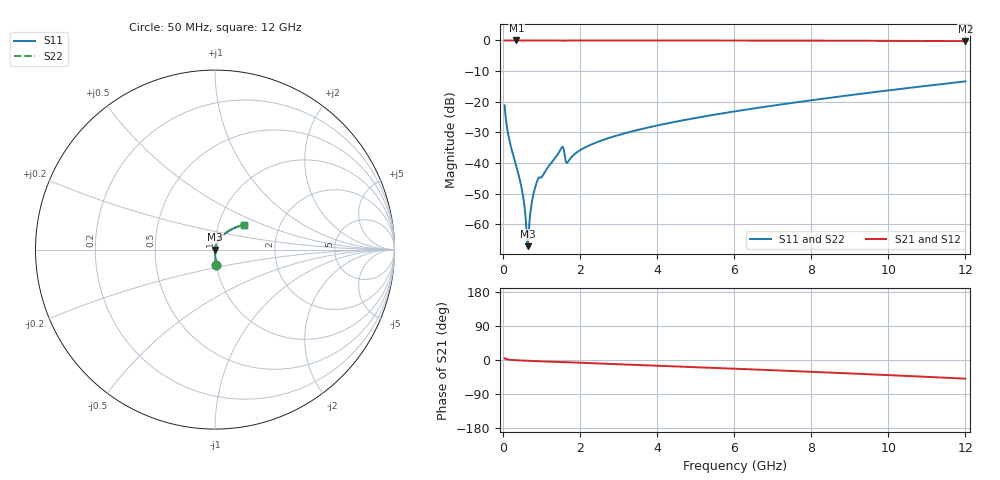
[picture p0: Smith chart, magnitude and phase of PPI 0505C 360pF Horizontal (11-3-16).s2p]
# MHz S MA R 50
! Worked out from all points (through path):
!   1601 points, 50 MHz to 12 GHz, reference 50 ohm
!   highest |S21| = 0.00 dB at 356.2 MHz (marker M1); lowest = -0.2 dB at 12 GHz (marker M2)
!   group delay of S21, straight-line fit = 11.4 ps
!   lowest |S11| = -67.1 dB at 647.5 MHz (marker M3), VSWR 1.00, Z = 50 - j0.00287 ohm
!   |S11| at or under -10 dB: start of sweep to end of sweep
!   |S22| runs from -67.1 to -13.4 dB; largest |S21 - S12| = 0
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50  0.08744 -85.0  0.996 4.9  0.996 4.9  0.08744 -85.0
176.9688  0.02312 -88.6  0.9994 0.8  0.9994 0.8  0.02312 -88.6
356.2188  0.008719 -88.4  0.9996 -0.6  0.9996 -0.6  0.008719 -88.4
498.125  0.003707 -85.3  0.9996 -1.4  0.9996 -1.4  0.003707 -85.3
550.4062  0.002319 -81.5  0.9996 -1.6  0.9996 -1.6  0.002319 -81.5
610.1562  0.0009463 -65.2  0.9995 -1.9  0.9995 -1.9  0.0009463 -65.2
647.5  0.0004392 -3.7  0.9995 -2.1  0.9995 -2.1  0.0004392 -3.7
684.8438  0.0009046 57.6  0.9995 -2.2  0.9995 -2.2  0.0009046 57.6
744.5938  0.002058 73.8  0.9995 -2.5  0.9995 -2.5  0.002058 73.8
796.875  0.003086 77.2  0.9994 -2.7  0.9994 -2.7  0.003086 77.2
864.0938  0.004447 77.7  0.9992 -3.0  0.9992 -3.0  0.004447 77.7
923.8438  0.005629 73.6  0.9986 -3.3  0.9986 -3.3  0.005629 73.6
1521.344  0.01751 68.7  0.9951 -5.8  0.9951 -5.8  0.01751 68.7
1558.688  0.01834 56.5  0.9913 -5.9  0.9913 -5.9  0.01834 56.5
1685.656  0.01029 65.2  0.9965 -5.9  0.9965 -5.9  0.01029 65.2
2044.156  0.01671 79.2  0.9988 -7.5  0.9988 -7.5  0.01671 79.2
2820.906  0.02638 77.7  0.9986 -10.5  0.9986 -10.5  0.02638 77.7
4038.312  0.04134 73.5  0.998 -15.2  0.998 -15.2  0.04134 73.5
6025  0.06965 66.1  0.9961 -23.0  0.9961 -23.0  0.06965 66.1
8019.156  0.106 58.1  0.9925 -31.2  0.9925 -31.2  0.106 58.1
10013.31  0.1534 49.5  0.986 -39.9  0.986 -39.9  0.1534 49.5
12000  0.2146 40.2  0.9741 -49.3  0.9741 -49.3  0.2146 40.2
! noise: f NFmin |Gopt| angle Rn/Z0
50  0.0003105  0.833  0.2438  0.0003923
1372  0.00391  0.6689  4.316  0.002265
2701  0.004976  0.5311  8.298  0.001862
4031  0.006474  0.4817  12.13  0.00211
5360  0.00798  0.4543  15.82  0.002409
6682  0.009473  0.4376  19.35  0.002721
8012  0.011  0.4282  22.74  0.00306
9341  0.01258  0.4248  25.99  0.003436
1.067e+04  0.01426  0.4264  29.12  0.003866
1.2e+04  0.01606  0.4327  32.13  0.004367
